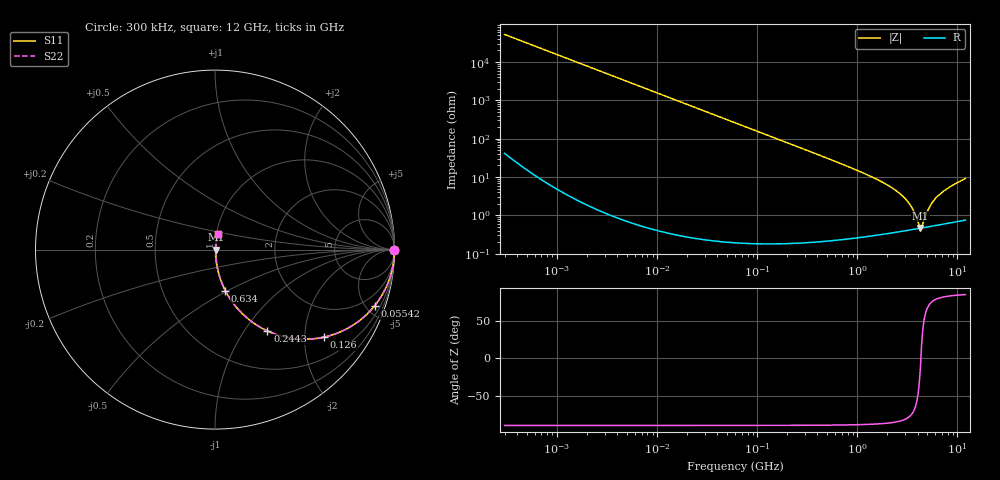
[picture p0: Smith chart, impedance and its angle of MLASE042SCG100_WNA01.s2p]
! MLASE042SCG100_WNA01  S-PARAMETER MODEL  ( General Type )
! Model Generated by TAIYO YUDEN Corporation (http://www.ty-top.com)
! Version 2.0
! TAIYO YUDEN Control No. 160513
! Copyright(c) 2013 TAIYO YUDEN CO.,LTD. All Rights Reserved.
! Product Description (link to TY-COMPAS)
! https://ds.yuden.co.jp/TYCOMPAS/or/detail?pn=MLASE042SCG100DWNA01&u=M
! Products Name : Multilayer Ceramic Capacitors
! Characteristics :
!  Capacitance : 10 pF , Rated Voltage : 16V , TCC : CG / C0G
!  Case Size : 0.4 x 0.2 / 0.016 x 0.008 [mm/inch] , Thickness : 0.2 / 0.008 [mm/inch]
!  (Conditions: Temperature = 25 degC , DC Bias Current/Voltage = 0A / 0V)
! External Node Assignments :
!  1  o---| |---o  2
! GND o---------o GND
! Frequency Range : 0.3MHz  -  12000MHz  [ 401 STEP ]
# MHz S RI R 50
! Freq[MHz].  S11 Real  S11 Imag  S21 Real  S21 Imag  S12 Real  S12 Imag  S22 Real  S22 Imag
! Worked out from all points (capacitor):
!   401 points, 300 kHz to 12 GHz, reference 50 ohm
!   read as one part in series: C = 10.1 pF near 316.3 kHz
!   lowest |Z| = 472 mohm at 4.271 GHz (marker M1)
!   series resonance near 4.313 GHz, so ESL is about 130 pH
!   S11 on the Smith chart (normalised r, x): 300 kHz: open; 55.42 MHz: 1.00, -5.67; 126 MHz: 1.00, -2.49; 244.3 MHz: 1.00, -1.28; 634 MHz: 1.00, -0.48; 12 GHz: 1.02, +0.18
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0.3  1 -0.00191  5.15e-06 0.00191  5.15e-06 0.00191  1 -0.00191
1.769972  0.9999 -0.0113  0.00013 0.0113  0.00013 0.0113  0.9999 -0.0113
10.44266  0.9956 -0.0662  0.00442 0.0662  0.00442 0.0662  0.9956 -0.0662
25.03118  0.9752 -0.1554  0.0248 0.1554  0.0248 0.1554  0.9752 -0.1554
55.41608  0.8891 -0.3137  0.1109 0.3137  0.1109 0.3137  0.8891 -0.3137
60  0.8724 -0.3333  0.1276 0.3333  0.1276 0.3333  0.8724 -0.3333
125.9782  0.6079 -0.4875  0.3921 0.4875  0.3921 0.4875  0.6079 -0.4875
244.3004  0.2916 -0.453  0.7084 0.453  0.7084 0.453  0.2916 -0.453
353.9943  0.1637 -0.3678  0.8363 0.3678  0.8363 0.3678  0.1637 -0.3678
634.0297  0.0574 -0.2279  0.9426 0.2279  0.9426 0.2279  0.0574 -0.2279
1296.429  0.0147 -0.1083  0.9853 0.1083  0.9853 0.1083  0.0147 -0.1083
2088.533  0.00667 -0.0571  0.9933 0.0571  0.9933 0.0571  0.00667 -0.0571
2650.866  0.00509 -0.0367  0.9949 0.0367  0.9949 0.0367  0.00509 -0.0367
3190.978  0.00454 -0.0223  0.9955 0.0223  0.9955 0.0223  0.00454 -0.0223
3547.679  0.00445 -0.0144  0.9956 0.0144  0.9956 0.0144  0.00445 -0.0144
4050.141  0.00452 -0.0048  0.9955 0.0048  0.9955 0.0048  0.00452 -0.0048
4270.516  0.0046 -0.000927  0.9954 0.000927  0.9954 0.000927  0.0046 -0.000927
4502.883  0.00473 0.00363  0.9953 -0.00363  0.9953 -0.00363  0.00473 0.00363
5278.635  0.00533 0.016  0.9947 -0.016  0.9947 -0.016  0.00533 0.016
6188.031  0.00631 0.0291  0.9937 -0.0291  0.9937 -0.0291  0.00631 0.0291
8281.503  0.00909 0.0529  0.9909 -0.0529  0.9909 -0.0529  0.00909 0.0529
12000  0.0155 0.0891  0.9845 -0.0891  0.9845 -0.0891  0.0155 0.0891
